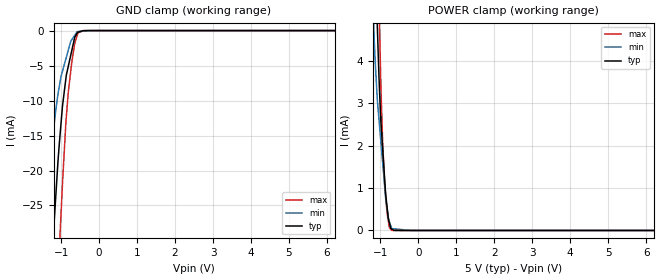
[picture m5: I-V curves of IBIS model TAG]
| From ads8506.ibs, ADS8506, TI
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|   tag Model
[Model]   TAG
Model_type   Input
Vinl = 0.8
Vinh = 2
|   typ   min   max
|   (nom PVT)   (Fast PVT)   (slow PVT)
|C_comp from frequency method(29MHz)
|Average
|C_comp   3.516e-12   2.967e-12   4.026e-12
|C_comp from LC tank measurement(L=1nH)
|Resonant Frequency(Hz)   3.270e+09   3.350e+09   3.230e+09
C_comp   2.371e-12   2.259e-12   2.430e-12
| Where nom  PVT is Nominal Process,  5V,  25C
|   Fast PVT is Strong Process,   5.25V,  -40C
|   Slow PVT is Weak Process,   4.75V,  85C
[Voltage Range]   5   4.75   5.25
|Ambient Temperature   25   85   -40
|Junction Temperature
[Temperature Range]   25   85   -40
[Power Clamp Reference]   5   4.75   5.25
[GND Clamp Reference]   0   0   0
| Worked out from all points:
|   GND clamp passes 1 mA (typ) near -0.64 V on its own axis
|   POWER clamp passes 1 mA (typ) near -0.87 V on its own axis
[GND Clamp]
|   Voltage   I(typ)   I(min)   I(max)
-5V       -471.6mA   -350.3mA   -579.3mA
-1.485V   -55.6mA    -30.2mA    -89.13mA
-1.306V   -37.91mA   -19.38mA   -64.46mA
-1.171V   -26.25mA   -12.8mA    -46.58mA
-1.05V    -16.31mA   -8.058mA   -31.59mA
-1.007V   -13.55mA   -6.68mA    -26.73mA
-882mV    -7.175mA   -4.19mA    -13.83mA
-813.7mV  -5.173mA   -2.847mA   -8.954mA
-719.2mV  -2.865mA   -1.297mA   -4.532mA
-574.7mV  -324.1uA   -139.9uA   -652.4uA
-383.2mV  -4.103uA   -70.28uA   -1.35uA
10V       0A         0A         0A
[POWER Clamp]
|   Voltage   I(typ)   I(min)   I(max)
-5V       185.4mA    155.9mA    225.8mA
-1.183V   8.759mA    4.973mA    12.36mA
-1.075V   4.71mA     3.041mA    7.149mA
-1.035V   3.611mA    2.614mA    5.369mA
-990mV    2.637mA    2.139mA    3.621mA
-939.7mV  1.948mA    1.608mA    2.115mA
-887.2mV  1.229mA    1.054mA    1.133mA
-865mV    923.9uA    818.8uA    882.3uA
-824.3mV  570.2uA    532.2uA    422.7uA
-761.2mV  183.4uA    203.3uA    66.2uA
-698.3mV  34.53uA    44.26uA    4.402uA
10V       0A         0A         0A
